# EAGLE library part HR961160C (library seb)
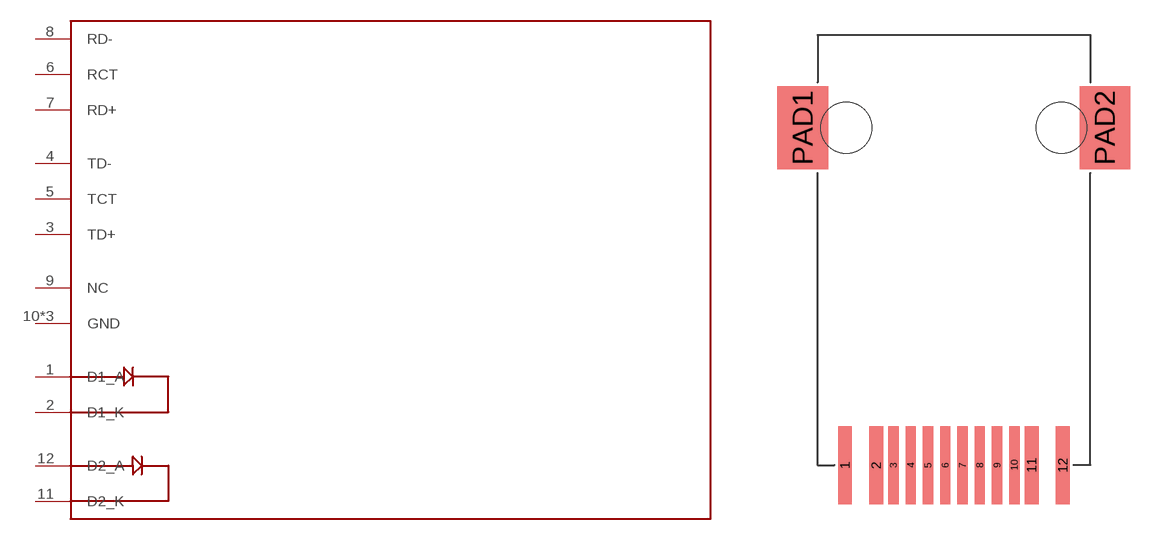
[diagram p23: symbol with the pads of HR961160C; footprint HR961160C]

Designator prefix -

## HR961160C  [HR961160C]
1  D1_A
2  D1_K
3  TD+
4  TD-
5  TCT
6  RCT
7  RD+
8  RD-
9  NC
10  GND
11  D2_K
12  D2_A
PAD1  GND
PAD2  GND

## Footprint HR961160C (pad centres in mm)
smd 0.81 x 4.6: 1 -6.43,0; 2 -4.59,0; 11 4.59,0; 12 6.43,0
smd 0.61 x 4.6: 3 -3.57,0; 4 -2.55,0; 5 -1.53,0; 6 -0.51,0; 7 0.51,0; 8 1.53,0; 9 2.55,0; 10 3.57,0
smd 3 x 4.9: PAD1 -8.92,19.92; PAD2 8.92,19.92
hole 3 at -6.35,19.92
hole 3 at 6.35,19.92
